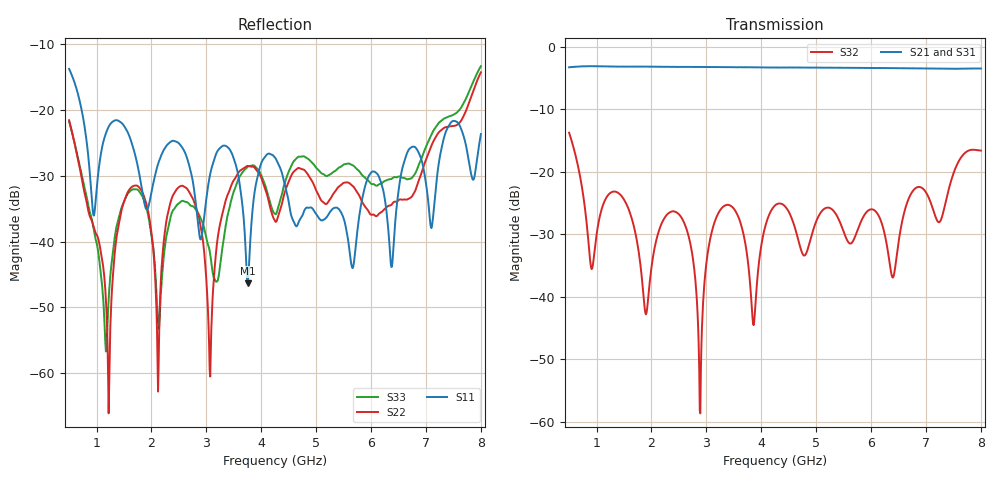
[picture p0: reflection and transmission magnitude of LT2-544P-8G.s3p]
! MTS Systemtechnik GmbH
! S-Parameters
! Model: LT2-544P-8G
! Rohde & Schwarz ZVB8 2Ports - Version 3.20 - 1145.1010k08 SN: 100119
! Converted & adapted with Octave
!		|  MTS  |
!		|  |--o OUT 2 (Port 3)
! C (Port 1) o--| LT2-544P-8G |
!		|  |--o OUT 1 (Port 2)
! S3P File: Measurements:
! <S11,S12,S13>,
! <S21,S22,S23>,
! <S31,S32,S33>:
# HZ  S  DB  R  50.00
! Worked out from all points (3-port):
!   751 points, 500 MHz to 8 GHz, reference 50 ohm
!   strongest paths, dB at 500 MHz, 2.37 GHz, 4.25 GHz, 6.13 GHz, 8 GHz:
!     S21: -3.3, -3.2, -3.4, -3.4, -3.5
!     S31: -3.3, -3.2, -3.4, -3.5, -3.6
!     S32: -13.8, -26.4, -25.4, -26.9, -16.6
!   lowest |S11| = -46.3 dB at 3.75 GHz (marker M1), VSWR 1.01, Z = 50.4 + j0.184 ohm
!   |S11| at or under -10 dB: start of sweep to end of sweep
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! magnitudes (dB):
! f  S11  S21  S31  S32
! 500 MHz  -13.8  -3.3  -3.3  -13.8
! 1.22 GHz  -22.5  -3.2  -3.2  -23.6
! 1.6 GHz  -24.0  -3.2  -3.2  -26.4
! 2.12 GHz  -28.2  -3.2  -3.2  -29.9
! 2.88 GHz  -39.3  -3.3  -3.3  -58.2
! 3.07 GHz  -29.7  -3.3  -3.3  -30.7
! 3.75 GHz  -46.3  -3.3  -3.3  -33.9
! 4.25 GHz  -27.2  -3.4  -3.4  -25.4
! 5.66 GHz  -44.0  -3.4  -3.5  -31.2
! 8 GHz  -23.7  -3.5  -3.6  -16.6
